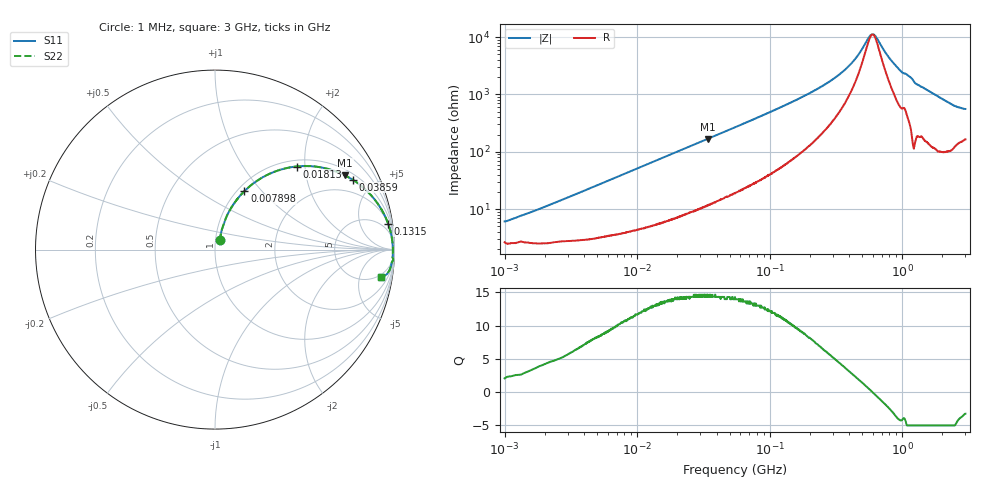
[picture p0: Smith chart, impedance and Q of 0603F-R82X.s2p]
!s-Parameter Generated by FASTRON Sdn. Bhd.
!FASTRON P/N : 0603F-R82X
!Keysight Technologies: E4991B_MY54100416_A.01.15
!Date: Wed Jun 19 15:32:15 2024
!Version  :Rev00  Wed Jun 19 15:32:15 2024
!Data & Calibration Information:
!Freq  S11  S21  S12  S22
!PortZ  Port1:50+j0  Port2:50+j0
!When reading reference impedance value at option line is always used.
! Remarks : This data is being provided solely for informational purposes.
# Hz S dB R 50
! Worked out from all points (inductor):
!   1601 points, 1 MHz to 3 GHz, reference 50 ohm
!   read as one part in series: L = 849 nH near 1.47 MHz
!   highest Q = 14.6 at 34.05 MHz (marker M1), where L = 784 nH
!   self-resonance near 597.4 MHz
!   S11 on the Smith chart (normalised r, x): 1 MHz: 1.05, +0.11; 7.898 MHz: 1.08, +0.81; 18.13 MHz: 1.13, +1.82; 38.59 MHz: 1.26, +3.79; 131.5 MHz: 2, +13; 3 GHz: 4, -11
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1000000  -24.50 61.2  -0.24 -3.1  -0.24 -3.1  -24.50 61.2
3804036  -14.40 70.8  -0.41 -10.9  -0.41 -10.9  -14.40 70.8
7898269  -8.76 63.3  -0.94 -21.3  -0.94 -21.3  -8.76 63.3
1.447069e7  -4.88 51.0  -2.17 -34.7  -2.17 -34.7  -4.88 51.0
1.812522e7  -3.74 45.4  -2.93 -40.4  -2.93 -40.4  -3.74 45.4
3.404917e7  -1.57 29.7  -6.08 -56.4  -6.08 -56.4  -1.57 29.7
3.858661e7  -1.30 26.9  -6.88 -59.1  -6.88 -59.1  -1.30 26.9
5.504702e7  -0.76 19.9  -9.35 -66.0  -9.35 -66.0  -0.76 19.9
1.314834e8  -0.22 8.6  -16.50 -76.2  -16.50 -76.2  -0.22 8.6
2.083556e8  -0.13 5.1  -21.00 -77.7  -21.00 -77.7  -0.13 5.1
2.884452e8  -0.10 3.2  -24.90 -76.5  -24.90 -76.5  -0.10 3.2
3.817355e8  -0.09 1.9  -29.30 -71.9  -29.30 -71.9  -0.09 1.9
4.548043e8  -0.08 1.1  -33.20 -63.7  -33.20 -63.7  -0.08 1.1
5.583748e8  -0.08 0.3  -39.80 -28.5  -39.80 -28.5  -0.08 0.3
5.899715e8  -0.08 0.1  -41.00 -6.1  -41.00 -6.1  -0.08 0.1
6.359588e8  -0.08 -0.3  -40.10 26.7  -40.10 26.7  -0.08 -0.3
7.925923e8  -0.08 -1.2  -33.00 66.0  -33.00 66.0  -0.08 -1.2
9.730857e8  -0.08 -2.1  -28.30 74.6  -28.30 74.6  -0.08 -2.1
1.11944e9  -0.08 -2.7  -26.50 77.8  -26.50 77.8  -0.08 -2.7
1.287806e9  -0.09 -3.7  -23.70 79.3  -23.70 79.3  -0.09 -3.7
2.371269e9  -0.29 -8.2  -16.80 72.6  -16.80 72.6  -0.29 -8.2
3e9  -0.56 -9.2  -15.50 63.6  -15.50 63.6  -0.56 -9.2
